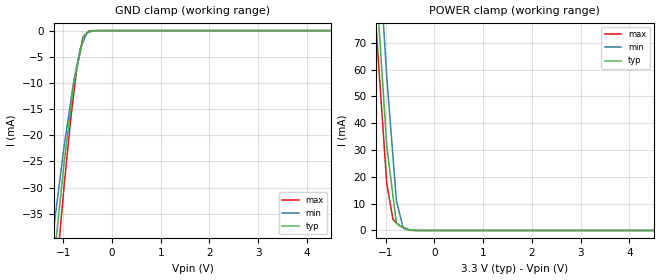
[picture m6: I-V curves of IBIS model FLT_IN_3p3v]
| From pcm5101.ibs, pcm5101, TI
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|   FLT_IN_3p3v
[Model]   FLT_IN_3p3v
Model_type   Input
Vinl = 0.99
Vinh = 2.31
|   typ   min   max
C_comp   1.387421673pF   1.361818132pF   1.403792289pF
[Voltage Range]   3.3   3   3.6
[Temperature Range]   27   105   -25
[Power Clamp Reference]   3.3   3   3.6
[GND Clamp Reference]   -0   -0   -0
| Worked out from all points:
|   GND clamp passes 1 mA (typ) near -0.58 V on its own axis
|   POWER clamp passes 1 mA (typ) near -0.63 V on its own axis
[GND Clamp]
|   Voltage   I(typ)   I(min)   I(max)
-3.3V     -527.4mA   -490.8mA   -553.6mA
-1.376V   -61.94mA   -52.32mA   -72.28mA
-1.178V   -42.72mA   -36.47mA   -50.11mA
-979.8mV  -24.99mA   -21.89mA   -29.39mA
-852.3mV  -15.29mA   -13.87mA   -17.38mA
-781.8mV  -9.934mA   -9.438mA   -11.84mA
-724.7mV  -7.371mA   -6.834mA   -7.349mA
-646.4mV  -3.858mA   -3.264mA   -3.625mA
-597.2mV  -1.648mA   -2.24mA    -1.282mA
-511mV    -520.4uA   -448.6uA   -446.7uA
-469.6mV  -219.9uA   -318.6uA   -45.44uA
6.6V      0A         0A         0A
[POWER Clamp]
|   Voltage   I(typ)   I(min)   I(max)
-3.3V     774.1mA    800.5mA    758.1mA
-1.376V   148.1mA    176.3mA    130.9mA
-1.178V   87.23mA    115.2mA    70.27mA
-979.8mV  31.54mA    57.35mA    17.54mA
-852.3mV  12.94mA    27.6mA     4.106mA
-781.8mV  2.67mA     11.17mA    2.884mA
-646.4mV  1.145mA    1.248mA    1.065mA
-583.8mV  440.6uA    769.8uA    491.1uA
-511mV    227.7uA    213.4uA    205.2uA
-240.2mV  18.36uA    663.8nA    484nA
6.6V      0A         0A         0A
